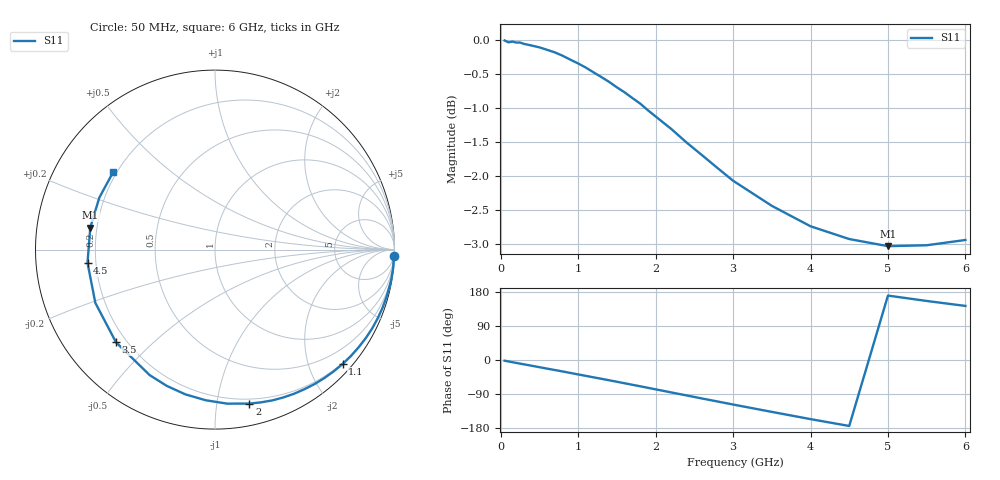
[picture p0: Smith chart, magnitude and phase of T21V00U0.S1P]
! SIEMENS Discrete & RF Semiconductors
! BAS70-04W
! Si Schottky Diode in SOT323
! VR = 1 V
! S-Parameters:  November  1997
# GHz  S  MA  R  50
!  f  S11
! GHz  MAG  ANG
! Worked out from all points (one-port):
!   34 points, 50 MHz to 6 GHz, reference 50 ohm
!   lowest |S11| = -3.0 dB at 5 GHz (marker M1), VSWR 5.79, Z = 8.7 + j4.24 ohm
!   |S11| at or under -10 dB: nowhere
!   S11 on the Smith chart (normalised r, x): 50 MHz: 0, -60; 1.1 GHz: 0.18, -2.60; 2 GHz: 0.16, -1.24; 3.5 GHz: 0.16, -0.39; 4.5 GHz: 0.17, -0.05; 6 GHz: 0.19, +0.33
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0.05  1 -1.9
0.15  0.9982 -5.8
0.25  0.9964 -9.6
0.4  0.9914 -15.2
0.5  0.9883 -19.0
0.6  0.9842 -22.8
0.7  0.9799 -26.5
0.8  0.9744 -30.3
1  0.9617 -38.1
1.1  0.9549 -41.9
1.2  0.9472 -45.8
1.4  0.9321 -53.5
1.6  0.9158 -61.4
1.7  0.907 -65.4
1.8  0.8985 -69.3
1.9  0.8884 -73.4
2  0.8791 -77.4
2.2  0.8609 -85.5
2.4  0.8411 -93.5
2.6  0.8232 -101.6
2.8  0.8054 -109.5
3  0.7884 -117.5
3.5  0.7555 -136.9
4  0.7298 -156.0
4.5  0.7141 -174.1
5  0.7056 170.0
5.5  0.7066 155.8
6  0.713 142.7
